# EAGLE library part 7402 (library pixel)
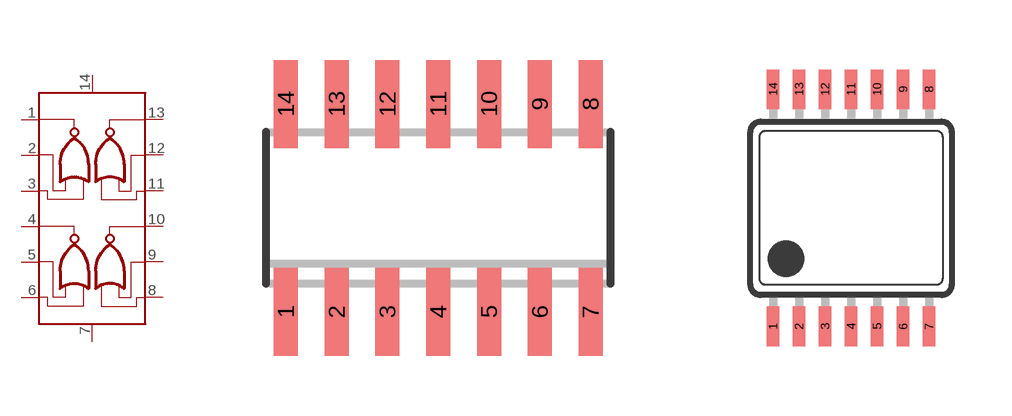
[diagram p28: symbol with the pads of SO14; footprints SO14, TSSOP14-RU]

Designator prefix -

## 7402  [SO14]
1  P$1
2  P$2
3  P$3
4  P$4
5  P$5
6  P$6
7  P$7
8  P$8
9  P$9
10  P$10
11  P$11
12  P$12
13  P$13
14  P$14

## 7402TSSOP14  [TSSOP14-RU]
Pads as for SO14

## Footprint SO14 (pad centres in mm)
14-Lead Narrow-Body SOIC (SO-14) Source: http://www.analog.com/static/imported-files/data_sheets/SSM2166.pdf
smd 0.6 x 2.2: 1 -3.81,-2.6; 2 -2.54,-2.6; 3 -1.27,-2.6; 4 0,-2.6; 5 1.27,-2.6; 6 2.54,-2.6; 7 3.81,-2.6; 8 3.81,2.6; 9 2.54,2.6; 10 1.27,2.6; 11 0,2.6; 12 -1.27,2.6; 13 -2.54,2.6; 14 -3.81,2.6

## Footprint TSSOP14-RU (pad centres in mm)
14-Lead Thin Shrink Small Outline Package [TSSOP] (RU-14) Source: www.analog.com .. OP1177_2177_4177.pdf
smd 0.305 x 0.991: 1 -1.95,-2.968; 2 -1.3,-2.968; 3 -0.65,-2.968; 4 0,-2.968; 5 0.65,-2.968; 6 1.3,-2.968; 7 1.95,-2.968; 8 1.95,2.968; 9 1.3,2.968; 10 0.65,2.968; 11 0,2.968; 12 -0.65,2.968; 13 -1.3,2.968; 14 -1.95,2.968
